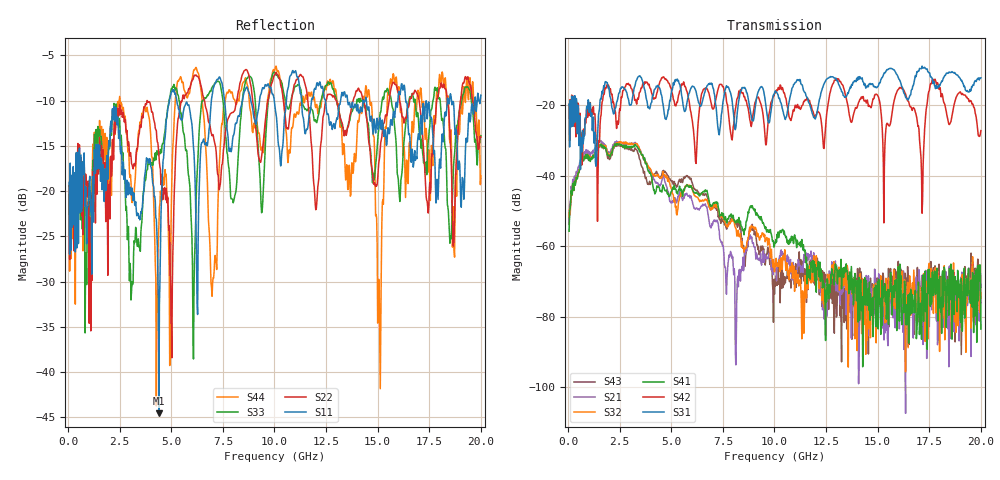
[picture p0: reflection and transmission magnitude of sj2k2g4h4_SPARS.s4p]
! FILE: E:\users\goganessyan\GBX_Backplane\FR408_backplane\1m_INBOUND_FEXT\sj2k2g4h4_SPARS.s4p
# MHZ S RI R 50.00
! FREQ  S11  S12  S13  S14
!  S21  S22  S23  S24
!  S31  S32  S33  S34
!  S41  S42  S43  S44
!  REAL  IMAG  REAL  IMAG  REAL  IMAG  REAL  IMAG
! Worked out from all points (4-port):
!   799 points, 50 MHz to 20 GHz, reference 50 ohm
!   strongest paths, dB at 50 MHz, 5.025 GHz, 10.03 GHz, 15.03 GHz, 20 GHz:
!     S31: -19.7, -15.7, -16.1, -14.6, -12.3
!     S42: -19.8, -16.3, -16.6, -17.5, -27.2
!     S41: -55.8, -44.3, -58.9, -83.5, -83.6
!     S32: -51.6, -44.0, -65.9, -76.6, -73.2
!     S21: -53.5, -47.8, -65.6, -73.2, -76.2
!     S43: -53.6, -41.7, -69.4, -82.5, -71.7
!   lowest |S11| = -44.5 dB at 4.4 GHz (marker M1), VSWR 1.01, Z = 50 + j0.593 ohm
!   |S11| at or under -10 dB: start of sweep to 4.909 GHz; 5.264 GHz to 6.943 GHz (1.678 GHz wide, 27.5 % of centre); 16.36 GHz to 18.37 GHz (2.005 GHz wide, 11.5 % of centre)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
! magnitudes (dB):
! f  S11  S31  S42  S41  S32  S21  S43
! 50 MHz  -19.0  -19.7  -19.8  -55.8  -51.6  -53.5  -53.6
! 4.4 GHz  -44.5  -14.9  -14.3  -43.3  -40.4  -42.5  -40.4
! 8.1 GHz  -12.6  -26.9  -21.3  -53.4  -54.7  -88.9  -53.3
! 14.5 GHz  -10.9  -14.4  -18.5  -76.8  -76.8  -83.8  -74.1
! 15.07 GHz  -12.5  -13.7  -18.5  -76.5  -74.4  -72.6  -76.9
! 15.7 GHz  -12.7  -9.7  -22.0  -79.6  -74.3  -78.4  -68.5
! 20 GHz  -9.4  -12.3  -27.2  -83.6  -73.2  -76.2  -71.7
